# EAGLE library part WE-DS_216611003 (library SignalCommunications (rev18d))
WE-DS D-SUB-Filter, Solder Pin Straight Characteristics Standard type filtered with 1000 pF High attenuation: max. ≥ 40 dB @ 180 MHz Choice of UNC 4/40 or through hole Rated voltage: 100 VDC Rated current @ 20 ºC: 5 A Withstand voltage: 250 VRMS Insulation resistance: min. 1000 MΩ Operating temperature: –55 ºC to +125 ºC Applications Filtering of interfaces External connection to -printer -sensor -display Details see: http://katalog.we-online.de/en/pbs/Filter_gerade Created on 2015-05-04 2015 (C) Wurth Elektronik
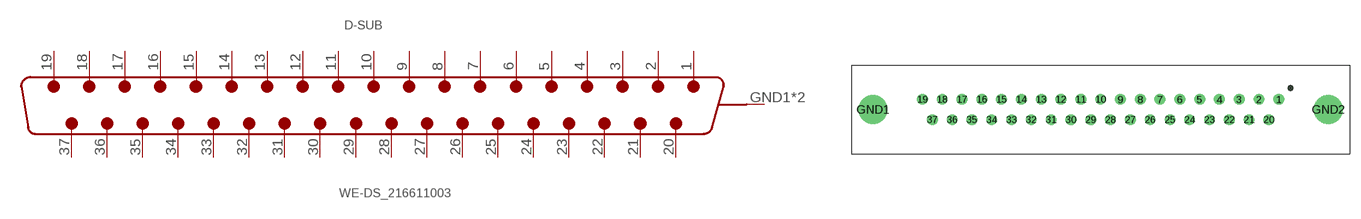
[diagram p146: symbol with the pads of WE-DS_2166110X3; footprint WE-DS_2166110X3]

Designator prefix D-SUB

## WE-DS_216611003 (WE-NUMBER: 216611003/37Pins_female)  [WE-DS_2166110X3]
1  19  pas
2  18  pas
3  17  pas
4  16  pas
5  15  pas
6  14  pas
7  13  pas
8  12  pas
9  11  pas
10  10  pas
11  9  pas
12  8  pas
13  7  pas
14  6  pas
15  5  pas
16  4  pas
17  3  pas
18  2  pas
19  1  pas
20  37  pas
21  36  pas
22  35  pas
23  34  pas
24  33  pas
25  32  pas
26  31  pas
27  30  pas
28  29  pas
29  28  pas
30  27  pas
31  26  pas
32  25  pas
33  24  pas
34  23  pas
35  22  pas
36  21  pas
37  20  pas
GND1  GND  pwr
GND2  GND  pwr

## Footprint WE-DS_2166110X3 (pad centres in mm)
drill 1: 1 24.84,1.42; 2 22.1,1.42; 3 19.33,1.42; 4 16.56,1.42; 5 13.82,1.42; 6 11.05,1.42; 7 8.28,1.42; 8 5.54,1.42; 9 2.77,1.42; 10 0,1.42; 11 -2.77,1.42; 12 -5.54,1.42; 13 -8.28,1.42; 14 -11.05,1.42; 15 -13.82,1.42; 16 -16.56,1.42; 17 -19.33,1.42; 18 -22.1,1.42; 19 -24.84,1.42; 20 23.47,-1.42; 21 20.7,-1.42; 22 17.96,-1.42; 23 15.19,-1.42; 24 12.42,-1.42; 25 9.68,-1.42; 26 6.91,-1.42; 27 4.14,-1.42; 28 1.38,-1.42; 29 -1.38,-1.42; 30 -4.14,-1.42; 31 -6.91,-1.42; 32 -9.68,-1.42; 33 -12.42,-1.42; 34 -15.19,-1.42; 35 -17.96,-1.42; 36 -20.7,-1.42; 37 -23.47,-1.42
drill 3: GND1 -31.75,0; GND2 31.75,0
